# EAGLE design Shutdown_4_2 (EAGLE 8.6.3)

## Sheet 1 of 5: Power
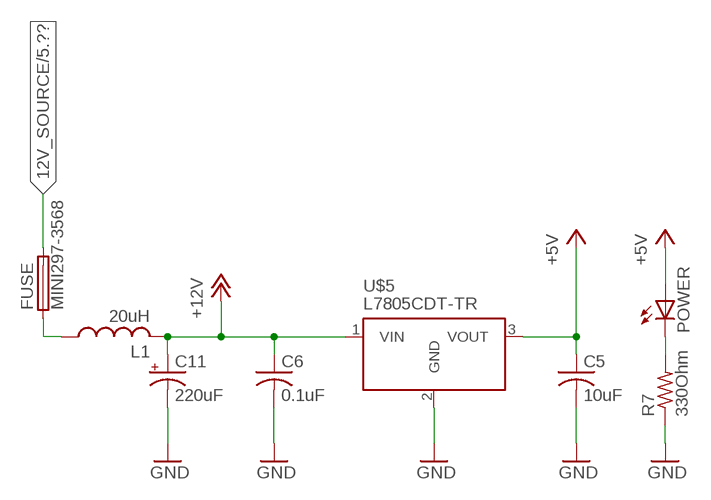
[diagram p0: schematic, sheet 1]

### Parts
C5  10uF  C0805  [C0805]
C6  0.1uF  C0805  [C0805]
C11  220uF  CPOL-USUD-6,3X7,7  [UD-6,3X7,7_NICHICON]
FUSE  MINI297-3568  [3568]
L1  20uH  MSS7348  [MSS7348]
POWER  LED0805  [LED0805]
R7  330Ohm  R0805  [R0805]
U$5  L7805CDT-TR  [DPACK]

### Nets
12V_SOURCE: FUSE.P$2 FUSE.P$3 ; also sheet 5
+5V: C5.1 POWER.1(A) U$5.3(VOUT) ; also sheet 2,3,5
+12V: C6.1 C11.+ L1.P$2 U$5.1(VIN) ; also sheet 3,4
GND: C5.2 C6.2 C11.- R7.1 U$5.2(GND) ; also sheet 2,3,4,5
N$2: FUSE.P$1 FUSE.P$4 L1.P$1
N$4: POWER.2(C) R7.2

## Sheet 2 of 5: Micro and CAN
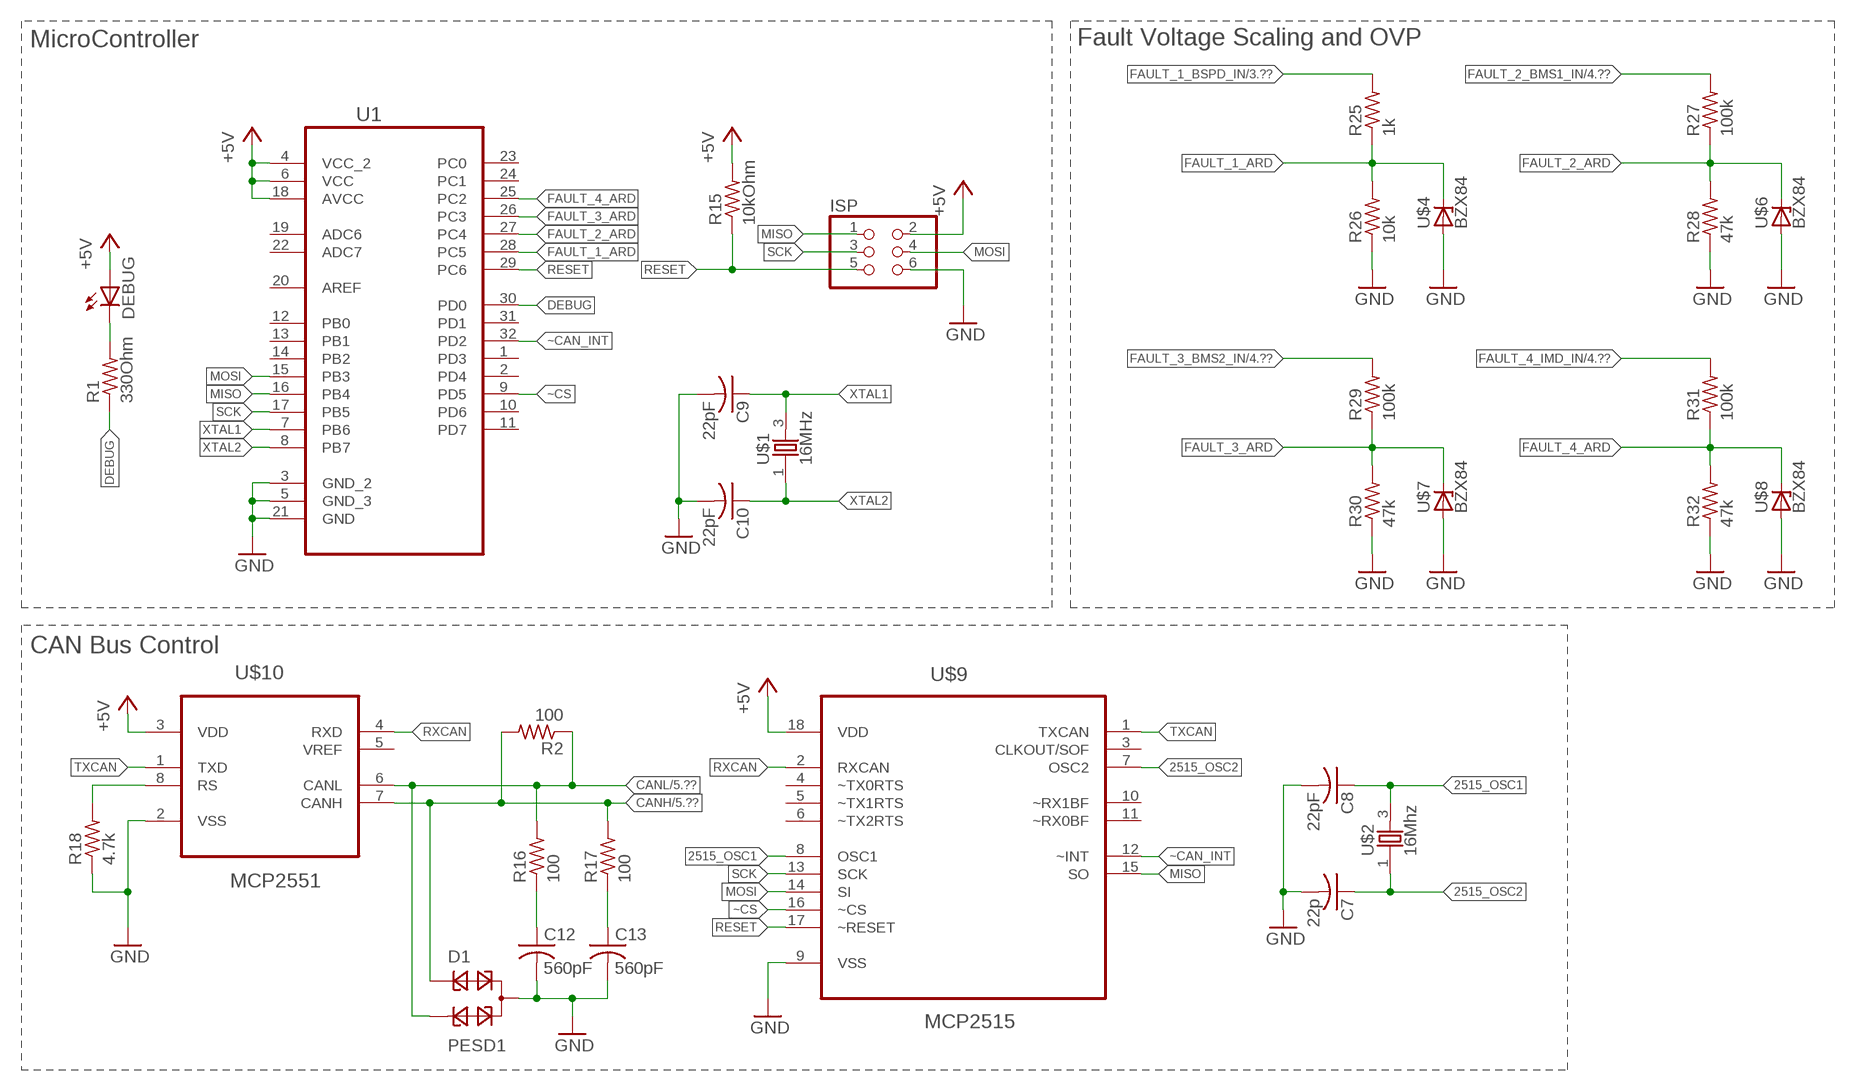
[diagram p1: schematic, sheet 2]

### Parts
C7  22p  C0805  [C0805]
C8  22pF  C0805  [C0805]
C9  22pF  C0805  [C0805]
C10  22pF  C0805  [C0805]
C12  560pF  C0805  [C0805]
C13  560pF  C0805  [C0805]
D1  PESD1  PESD1CAN  [SOT23]
DEBUG  LED0805  [LED0805]
ISP  PINHD-2X3  [2X03]
R1  330Ohm  R0805  [R0805]
R2  100  R0805  [R0805]
R15  10kOhm  R0805  [R0805]
R16  100  R0805  [R0805]
R17  100  R0805  [R0805]
R18  4.7k  R0805  [R0805]
R25  1k  R0805  [R0805]
R26  10k  R0805  [R0805]
R27  100k  R0805  [R0805]
R28  47k  R0805  [R0805]
R29  100k  R0805  [R0805]
R30  47k  R0805  [R0805]
R31  100k  R0805  [R0805]
R32  47k  R0805  [R0805]
U1  ATMEGA328P-AU  [QFP80P900X900X120-32N]
U$1  16MHz  406CYRYSTAL  [CTS406]
U$2  16Mhz  406CYRYSTAL  [CTS406]
U$4  BZX84  [SOT23]
U$6  BZX84  [SOT23]
U$7  BZX84  [SOT23]
U$8  BZX84  [SOT23]
U$9  MCP2515  MCP2515-I/SO  [SOIC127P1034X264-18N]
U$10  MCP2551  MCP2551-I/SN  [SOIC127P600X175-8N]

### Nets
2515_OSC1: C8.1 U$2.3 U$9.8(OSC1)
2515_OSC2: C7.1 U$2.1 U$9.7(OSC2)
+5V: DEBUG.1(A) ISP.2 R15.2 U1.4(VCC_2) U1.6(VCC) U1.18(AVCC) U$9.18(VDD) U$10.3(VDD) ; also sheet 1,3,5
CANH: D1.1 R2.2 R17.2 U$10.7(CANH) ; also sheet 5
CANL: D1.2 R2.1 R16.2 U$10.6(CANL) ; also sheet 5
DEBUG: R1.1 U1.30(PD0)
FAULT_1_ARD: R25.1 R26.2 U1.28(PC5) U$4.3(C)
FAULT_1_BSPD_IN: R25.2 ; also sheet 3,4
FAULT_2_ARD: R27.1 R28.2 U1.27(PC4) U$6.3(C)
FAULT_2_BMS1_IN: R27.2 ; also sheet 4,5
FAULT_3_ARD: R29.1 R30.2 U1.26(PC3) U$7.3(C)
FAULT_3_BMS2_IN: R29.2 ; also sheet 4,5
FAULT_4_ARD: R31.1 R32.2 U1.25(PC2) U$8.3(C)
FAULT_4_IMD_IN: R31.2 ; also sheet 4,5
GND: C7.2 C8.2 C9.2 C10.2 C12.2 C13.2 D1.3 ISP.6 R18.1 R26.1 R28.1 R30.1 R32.1 U1.3(GND_2) U1.5(GND_3) U1.21(GND) U$4.1(A) U$6.1(A) U$7.1(A) U$8.1(A) U$9.9(VSS) U$10.2(VSS) ; also sheet 1,3,4,5
MISO: ISP.1 U1.16(PB4) U$9.15(SO)
MOSI: ISP.4 U1.15(PB3) U$9.14(SI)
N$1: DEBUG.2(C) R1.2
N$12: C12.1 R16.1
N$13: C13.1 R17.1
N$14: R18.2 U$10.8(RS)
RESET: ISP.5 R15.1 U1.29(PC6) U$9.17(~RESET)
RXCAN: U$9.2(RXCAN) U$10.4(RXD)
SCK: ISP.3 U1.17(PB5) U$9.13(SCK)
TXCAN: U$9.1(TXCAN) U$10.1(TXD)
XTAL1: C9.1 U1.7(PB6) U$1.3
XTAL2: C10.1 U1.8(PB7) U$1.1
~CAN_INT: U1.32(PD2) U$9.12(~INT)
~CS: U1.9(PD5) U$9.16(~CS)
Unconnected: U1.1(PD3) U1.2(PD4) U1.10(PD6) U1.11(PD7) U1.12(PB0) U1.13(PB1) U1.14(PB2) U1.19(ADC6) U1.20(AREF) U1.22(ADC7) U1.23(PC0) U1.24(PC1) U1.31(PD1) U$9.3(CLKOUT/SOF) U$9.4(~TX0RTS) U$9.5(~TX1RTS) U$9.6(~TX2RTS) U$9.10(~RX1BF) U$9.11(~RX0BF) U$10.5(VREF)

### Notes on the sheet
- MicroController | Fault Voltage Scaling and OVP
- CAN Bus Control

## Sheet 3 of 5: BSPD Detection Circuit
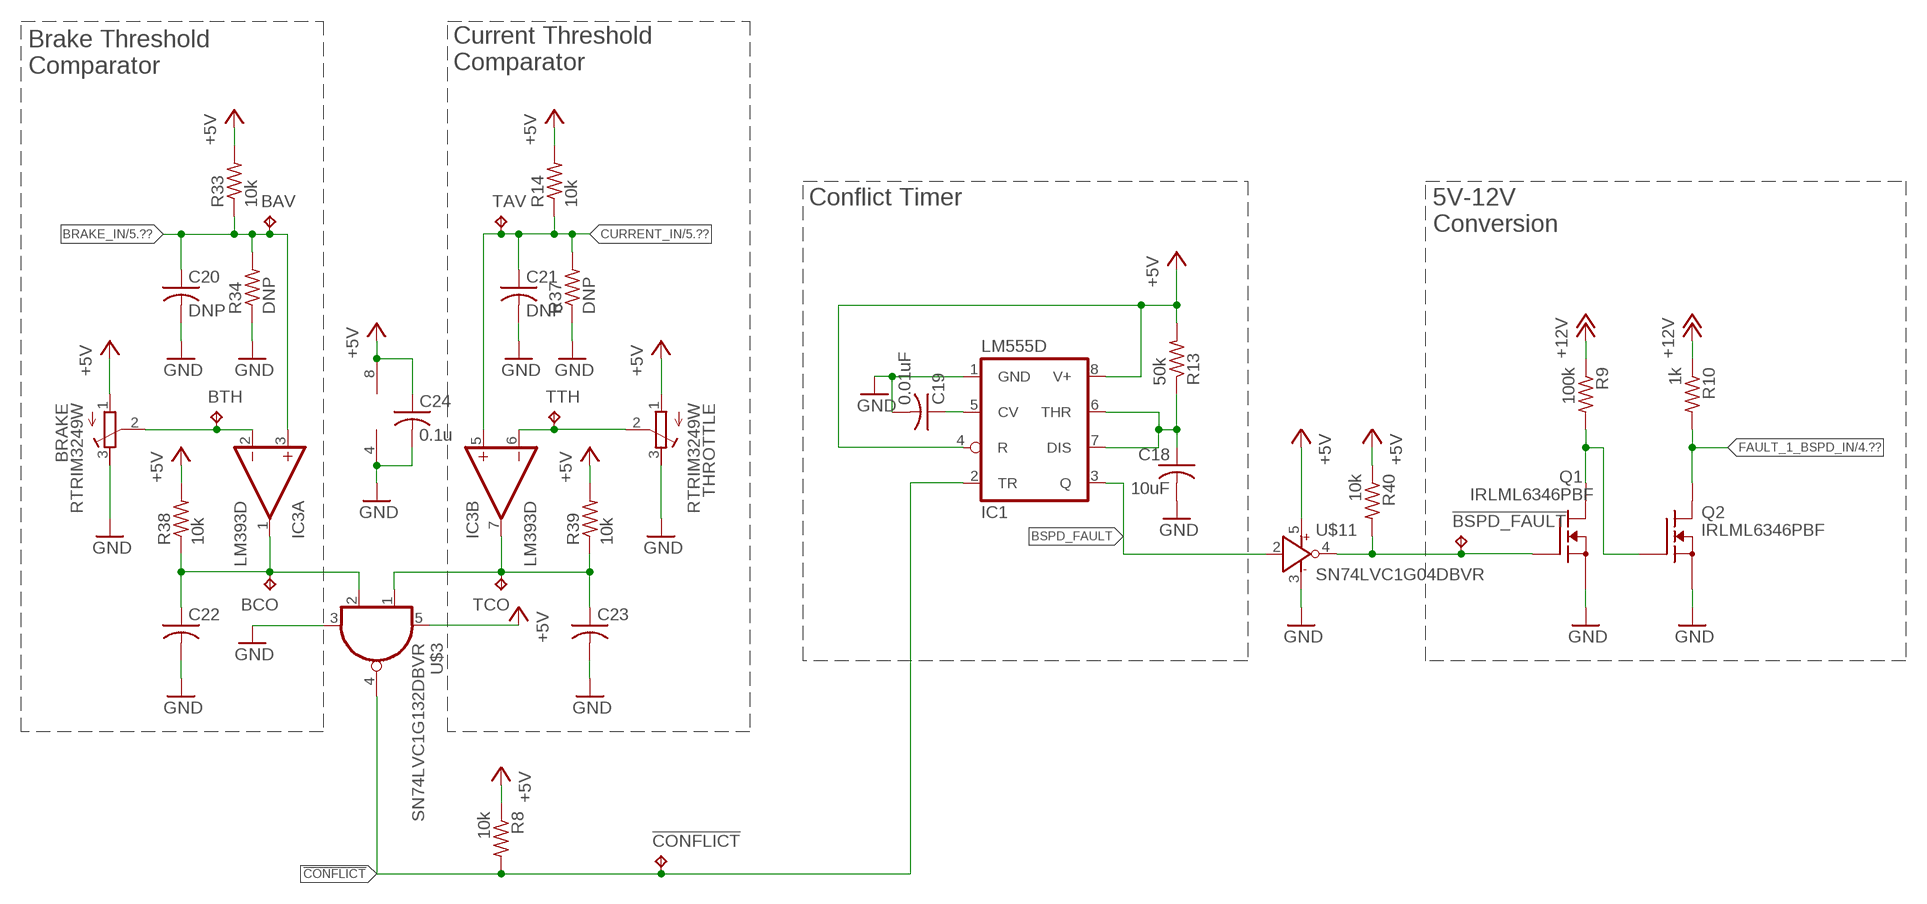
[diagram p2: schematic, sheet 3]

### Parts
!BSPD_FAULT  TPTP09R  [TP09R]
!CONFLICT  TPTP09R  [TP09R]
BAV  TPTP09R  [TP09R]
BCO  TPTP09R  [TP09R]
BRAKE  RTRIM3249W  [RTRIM3299W]
BTH  TPTP09R  [TP09R]
C18  10uF  C0805  [C0805]
C19  0.01uF  C0805  [C0805]
C20  DNP  C0805  [C0805]
C21  DNP  C0805  [C0805]
C22  C0805  [C0805]
C23  C0805  [C0805]
C24  0.1u  C0805  [C0805]
IC1  LM555D  [SO08]
IC3  LM393D  [SO08]
Q1  IRLML6346PBF  [SOT23]
Q2  IRLML6346PBF  [SOT23]
R8  10k  R0805  [R0805]
R9  100k  R0805  [R0805]
R10  1k  R0805  [R0805]
R13  50k  R0805  [R0805]
R14  10k  R0805  [R0805]
R33  10k  R0805  [R0805]
R34  DNP  R0805  [R0805]
R37  DNP  R0805  [R0805]
R38  10k  R0805  [R0805]
R39  10k  R0805  [R0805]
R40  10k  R0805  [R0805]
TAV  TPTP09R  [TP09R]
TCO  TPTP09R  [TP09R]
THROTTLE  RTRIM3249W  [RTRIM3299W]
TTH  TPTP09R  [TP09R]
U$3  SN74LVC1G132DBVR  [SOT23-5L]
U$11  SN74LVC1G04DBVR  [SOT23-5L]

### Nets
!CONFLICT: !CONFLICT.TP IC1.2(TR) R8.2 U$3.4(Y)
+5V: BRAKE.1(A) C24.1 IC1.4(R) IC1.8(V+) IC3.8(P:V+) R8.1 R13.2 R14.2 R33.2 R38.2 R39.2 R40.1 THROTTLE.1(A) U$3.5(V+) U$11.5(V+) ; also sheet 1,2,5
+12V: R9.1 R10.1 ; also sheet 1,4
BRAKE_IN: BAV.TP C20.1 IC3.3(A:+IN) R33.1 R34.2 ; also sheet 5
BSPD_FAULT: IC1.3(Q) U$11.2(A)
CURRENT_IN: C21.1 IC3.5(B:+IN) R14.1 R37.2 TAV.TP ; also sheet 5
FAULT_1_BSPD_IN: Q2.3(D) R10.2 ; also sheet 2,4
GND: BRAKE.3(E) C18.2 C19.2 C20.2 C21.2 C22.2 C23.2 C24.2 IC1.1(GND) IC3.4(P:V-) Q1.2(S) Q2.2(S) R34.1 R37.1 THROTTLE.3(E) U$3.3(GND) U$11.3(GND) ; also sheet 1,2,4,5
N$3: C23.1 IC3.7(B:OUT) R39.1 TCO.TP U$3.1(A)
N$5: BCO.TP C22.1 IC3.1(A:OUT) R38.1 U$3.2(B)
N$6: BRAKE.2(S) BTH.TP IC3.2(A:-IN)
N$7: !BSPD_FAULT.TP Q1.1(G) R40.2 U$11.4(Y)
N$10: C18.1 IC1.6(THR) IC1.7(DIS) R13.1
N$11: C19.1 IC1.5(CV)
N$15: Q1.3(D) Q2.1(G) R9.2
N$16: IC3.6(B:-IN) THROTTLE.2(S) TTH.TP

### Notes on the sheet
- Current Threshold
  Comparator
- Brake Threshold
  Comparator
- Conflict Timer
- 5V-12V
  Conversion

## Sheet 4 of 5: AIR Shutdown Relays + Fault Indication
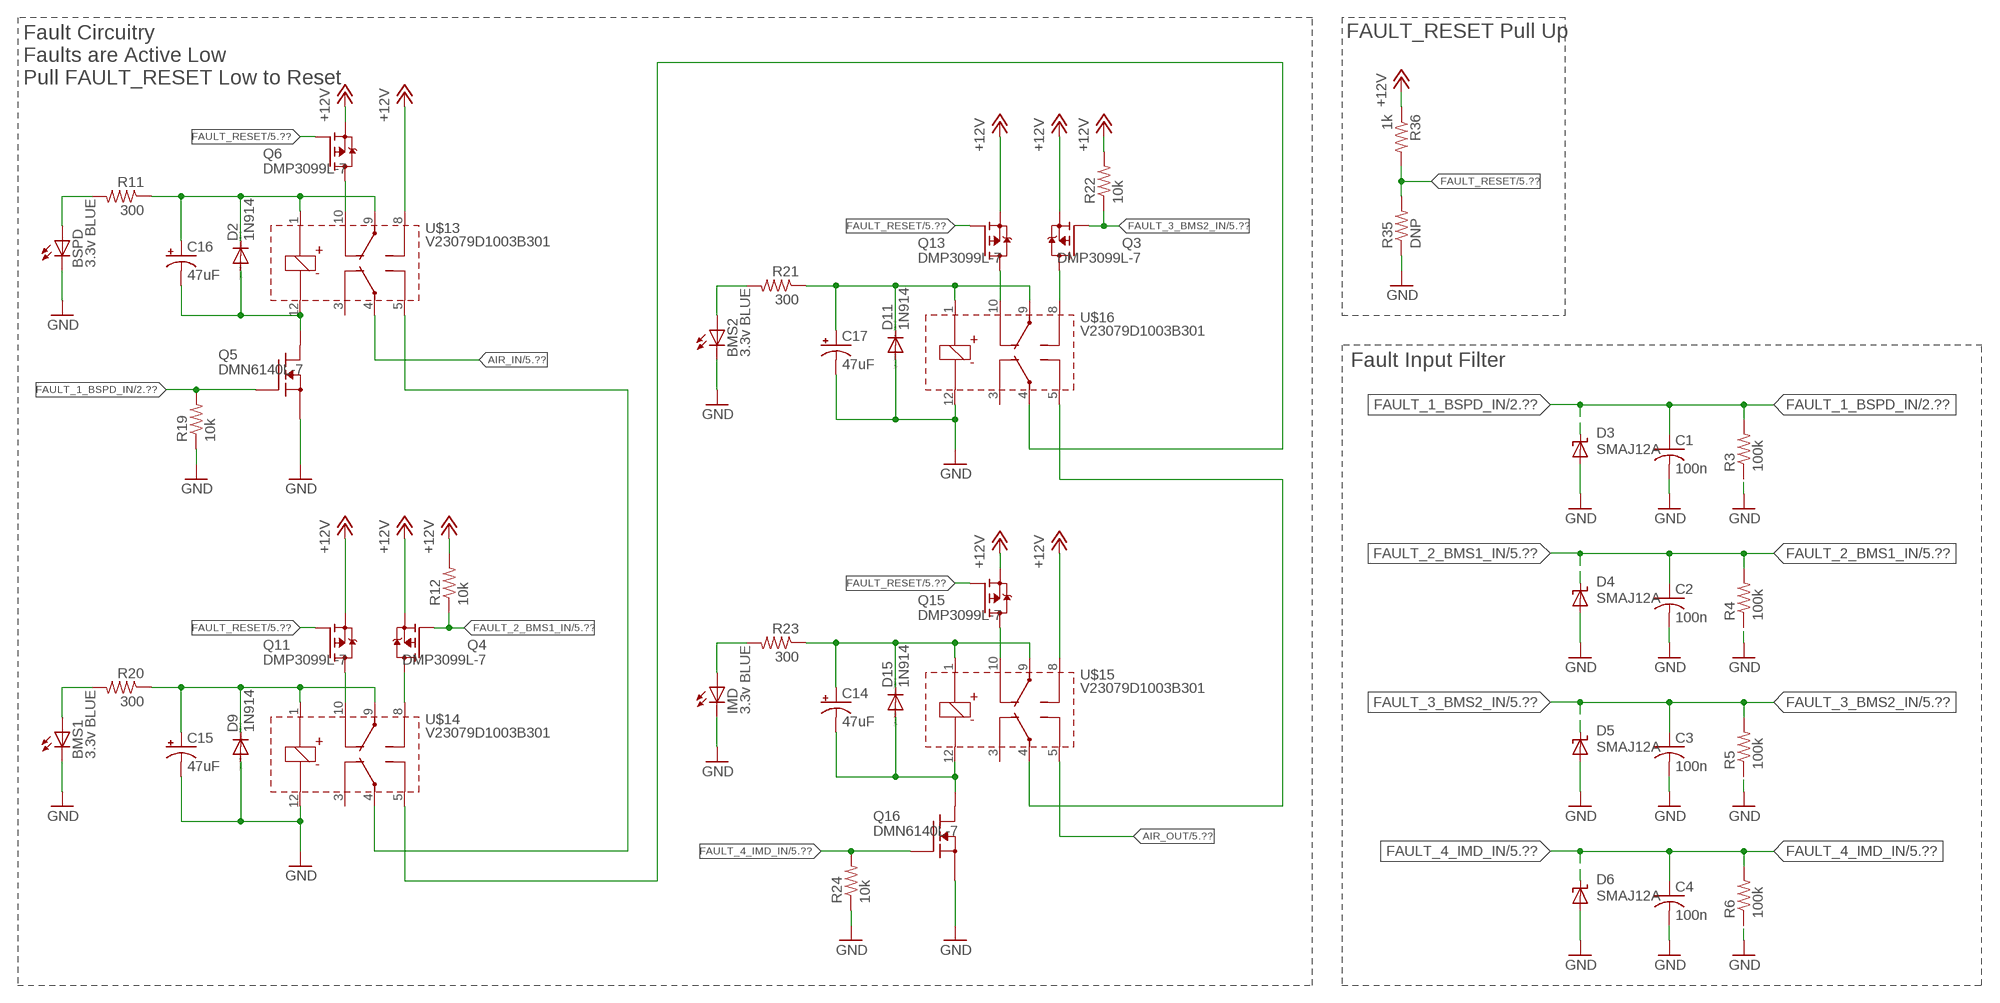
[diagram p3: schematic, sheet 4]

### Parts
BMS1  3.3v BLUE  LEDCHIPLED_0805  [CHIPLED_0805]
BMS2  3.3v BLUE  LEDCHIPLED_0805  [CHIPLED_0805]
BSPD  3.3v BLUE  LEDCHIPLED_0805  [CHIPLED_0805]
C1  100n  C0805  [C0805]
C2  100n  C0805  [C0805]
C3  100n  C0805  [C0805]
C4  100n  C0805  [C0805]
C14  47uF  CPOL-USUD-6,3X5,8  [UD-6,3X5,8_NICHICON]
C15  47uF  CPOL-USUD-6,3X5,8  [UD-6,3X5,8_NICHICON]
C16  47uF  CPOL-USUD-6,3X5,8  [UD-6,3X5,8_NICHICON]
C17  47uF  CPOL-USUD-6,3X5,8  [UD-6,3X5,8_NICHICON]
D2  1N914  [SOD323-F]
D3  SMAJ12A  [DO-214AC]
D4  SMAJ12A  [DO-214AC]
D5  SMAJ12A  [DO-214AC]
D6  SMAJ12A  [DO-214AC]
D9  1N914  [SOD323-F]
D11  1N914  [SOD323-F]
D15  1N914  [SOD323-F]
IMD  3.3v BLUE  LEDCHIPLED_0805  [CHIPLED_0805]
Q3  DMP3099L-7  [SOT23]
Q4  DMP3099L-7  [SOT23]
Q5  DMN6140L-7  [SOT23]
Q6  DMP3099L-7  [SOT23]
Q11  DMP3099L-7  [SOT23]
Q13  DMP3099L-7  [SOT23]
Q15  DMP3099L-7  [SOT23]
Q16  DMN6140L-7  [SOT23]
R3  100k  R0805  [R0805]
R4  100k  R0805  [R0805]
R5  100k  R0805  [R0805]
R6  100k  R0805  [R0805]
R11  300  R0805  [R0805]
R12  10k  R0805  [R0805]
R19  10k  R0805  [R0805]
R20  300  R0805  [R0805]
R21  300  R0805  [R0805]
R22  10k  R0805  [R0805]
R23  300  R0805  [R0805]
R24  10k  R0805  [R0805]
R35  DNP  R0805  [R0805]
R36  1k  R0805  [R0805]
U$13  V23079D1003B301  [DPDT_2C]
U$14  V23079D1003B301  [DPDT_2C]
U$15  V23079D1003B301  [DPDT_2C]
U$16  V23079D1003B301  [DPDT_2C]

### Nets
+12V: Q3.2(S) Q4.2(S) Q6.2(S) Q11.2(S) Q13.2(S) Q15.2(S) R12.2 R22.2 R36.1 U$13.8(2_ACTIVE) U$15.8(2_ACTIVE) ; also sheet 1,3
AIR_IN: U$13.4(1_CENTER) ; also sheet 5
AIR_OUT: U$15.5(1_ACTIVE) ; also sheet 5
BMS1_FAULT_INDICATOR: C15.+ D9.C R20.1 U$14.1(COIL+) U$14.9(2_CENTER)
BMS2_FAULT_INDICATOR: C17.+ D11.C R21.1 U$16.1(COIL+) U$16.9(2_CENTER)
BSPD_FAULT_INDICATOR: C16.+ D2.C R11.1 U$13.1(COIL+) U$13.9(2_CENTER)
FAULT_1_BSPD_IN: C1.1 D3.C Q5.1(G) R3.2 R19.2 ; also sheet 2,3
FAULT_2_BMS1_IN: C2.1 D4.C Q4.1(G) R4.2 R12.1 ; also sheet 2,5
FAULT_3_BMS2_IN: C3.1 D5.C Q3.1(G) R5.2 R22.1 ; also sheet 2,5
FAULT_4_IMD_IN: C4.1 D6.C Q16.1(G) R6.2 R24.2 ; also sheet 2,5
FAULT_RESET: Q6.1(G) Q11.1(G) Q13.1(G) Q15.1(G) R35.2 R36.2 ; also sheet 5
GND: BMS1.C BMS2.C BSPD.C C1.2 C2.2 C3.2 C4.2 C15.- C17.- D3.A D4.A D5.A D6.A D9.A D11.A IMD.C Q5.2(S) Q16.2(S) R3.1 R4.1 R5.1 R6.1 R19.1 R24.1 R35.1 U$14.12(COIL-) U$16.12(COIL-) ; also sheet 1,2,3,5
IMD_FAULT_INDICATOR: C14.+ D15.C R23.1 U$15.1(COIL+) U$15.9(2_CENTER)
N$8: BSPD.A R11.2
N$9: Q4.3(D) U$14.8(2_ACTIVE)
N$18: Q3.3(D) U$16.8(2_ACTIVE)
N$27: U$13.5(1_ACTIVE) U$14.4(1_CENTER)
N$28: Q6.3(D) U$13.10(2_REST)
N$31: U$14.5(1_ACTIVE) U$16.4(1_CENTER)
N$32: C16.- D2.A Q5.3(D) U$13.12(COIL-)
N$34: BMS1.A R20.2
N$35: Q11.3(D) U$14.10(2_REST)
N$36: U$15.4(1_CENTER) U$16.5(1_ACTIVE)
N$37: BMS2.A R21.2
N$38: Q13.3(D) U$16.10(2_REST)
N$42: IMD.A R23.2
N$43: Q15.3(D) U$15.10(2_REST)
N$44: C14.- D15.A Q16.3(D) U$15.12(COIL-)
Unconnected: U$13.3(1_REST) U$14.3(1_REST) U$15.3(1_REST) U$16.3(1_REST)

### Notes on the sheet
- FAULT_RESET Pull Up
- Fault Circuitry
  Faults are Active Low
  Pull FAULT_RESET Low to Reset
- Fault Input Filter

## Sheet 5 of 5: Connector
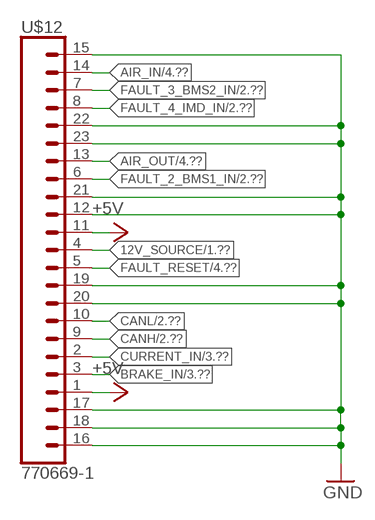
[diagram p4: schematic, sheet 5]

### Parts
U$12  770669-1  [770669-1]

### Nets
12V_SOURCE: U$12.4 ; also sheet 1
+5V: U$12.1 U$12.11 ; also sheet 1,2,3
AIR_IN: U$12.14 ; also sheet 4
AIR_OUT: U$12.13 ; also sheet 4
BRAKE_IN: U$12.3 ; also sheet 3
CANH: U$12.9 ; also sheet 2
CANL: U$12.10 ; also sheet 2
CURRENT_IN: U$12.2 ; also sheet 3
FAULT_2_BMS1_IN: U$12.6 ; also sheet 2,4
FAULT_3_BMS2_IN: U$12.7 ; also sheet 2,4
FAULT_4_IMD_IN: U$12.8 ; also sheet 2,4
FAULT_RESET: U$12.5 ; also sheet 4
GND: U$12.12 U$12.15 U$12.16 U$12.17 U$12.18 U$12.19 U$12.20 U$12.21 U$12.22 U$12.23 ; also sheet 1,2,3,4

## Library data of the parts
!BSPD_FAULT !CONFLICT BAV BCO BTH TAV TCO TTH = testpad:TP: Test pad
BMS1 BMS2 BSPD IMD = led:LED: LED
BRAKE THROTTLE = Resistors:RTRIM3249W
C1-C10 C12 C13 C18-C24 = Capacitors:C0805
C11 C14-C17 = rcl:CPOL-US: POLARIZED CAPACITOR, American symbol; SPICEPREFIX: C
D1 = diode:PESD1CAN: CAN bus ESD protection diode Source: http://www.nxp.com/documents/data_sheet/PESD1CAN.pdf
D2 D9 D11 D15 = Diodes:1N914
D3-D6 = Diodes:SMAJ12A
DEBUG POWER = LEDS:LED0805
FUSE = Fuse:MINI297-3568
IC1 = bspd2:*555: TIMER Changed DIP package to have round (not oval) pin pads http://www.ladyada.net/library/pcb/eaglelibrary.html
IC3 = IC's:LM393: COMPARATOR
ISP = pinhead:PINHD-2X3: PIN HEADER
L1 = Inductors:MSS7348
Q1 Q2 = TRANS:IRLML6346PBF: IRLML6346TRPBF Vgs(th) = 1.1V, Rds(on) = 63 mOhm, Vds(max) = 30V
Q3 Q4 Q6 Q11 Q13 Q15 = TRANS:DMP3099L-7: DMP3099L-7 P-Channel Vgs(th) = 2.1V, Rds(on) = 64 mohm, Vds(max) = 30V
Q5 Q16 = TRANS:DMN6140L-7: DMN6140L-7 Vgs(th) = 3V, Rds(on) = 140mOhm, Vds(max) = 60V
R1-R40 = Resistors:R0805
U1 = Atmel_By_element14_Batch_1-00:ATMEGA328P-AU: 8-bit Microcontroller with In-System Programmable Flash; MPN: ATMEGA328P-AU; OC_FARNELL: 1715486; OC_NEWARK: 14R4631; PACKAGE: TQFP-32; SUPPLIER: Atmel
U$1 U$2 = Display_Custom:406CYRYSTAL: Crystal Oscillator in 406 SMT Package
U$3 = Display_Custom:SN74LVC1G132DBVR: TI Single NAND SN74LVC1G132DBVR http://www.ti.com/lit/ds/symlink/sn74lvc1g132.pdf
U$4 U$6-U$8 = Diodes:BZX84: Zener Diode
U$5 = Display_Custom:L7805CDT-TR: ST - L78 L7805CDT-TR 5V 1.5A Linear Regulator
U$9 = Microchip_By_element14_Batch_1:MCP2515-I/SO: CAN Controller; MPN: MCP2515-I/SO; OC_FARNELL: 1292239; OC_NEWARK: 29H7136; PACKAGE: SOIC-18; SUPPLIER: Microchip
U$10 = Microchip_By_element14_Batch_1:MCP2551-I/SN: High-Speed CAN Transceiver; MPN: MCP2551-I/SN; OC_FARNELL: 9758569; OC_NEWARK: 69K7604; PACKAGE: SOIC-8; SUPPLIER: Microchip
U$11 = Display_Custom:SN74LVC1G04DBVR: TI Single Chip Inverter SN74LVC1G04DBVR http://www.ti.com/lit/ds/symlink/sn74lvc1g04.pdf
U$12 = IFE_AMPSEAL_Conn:770669-1: AMPSEAL 23pin Connector Ampseal 23-pin connector Model: 770669-1
U$13-U$16 = Display_Custom:V23079D1003B301: TE Connectivity Potter & Brumfield Relays V23079D1003B301 http://www.te.com/commerce/DocumentDelivery/DDEController?Action=srchrtrv&DocNm=108-98002&DocType=SS&DocLang=EN

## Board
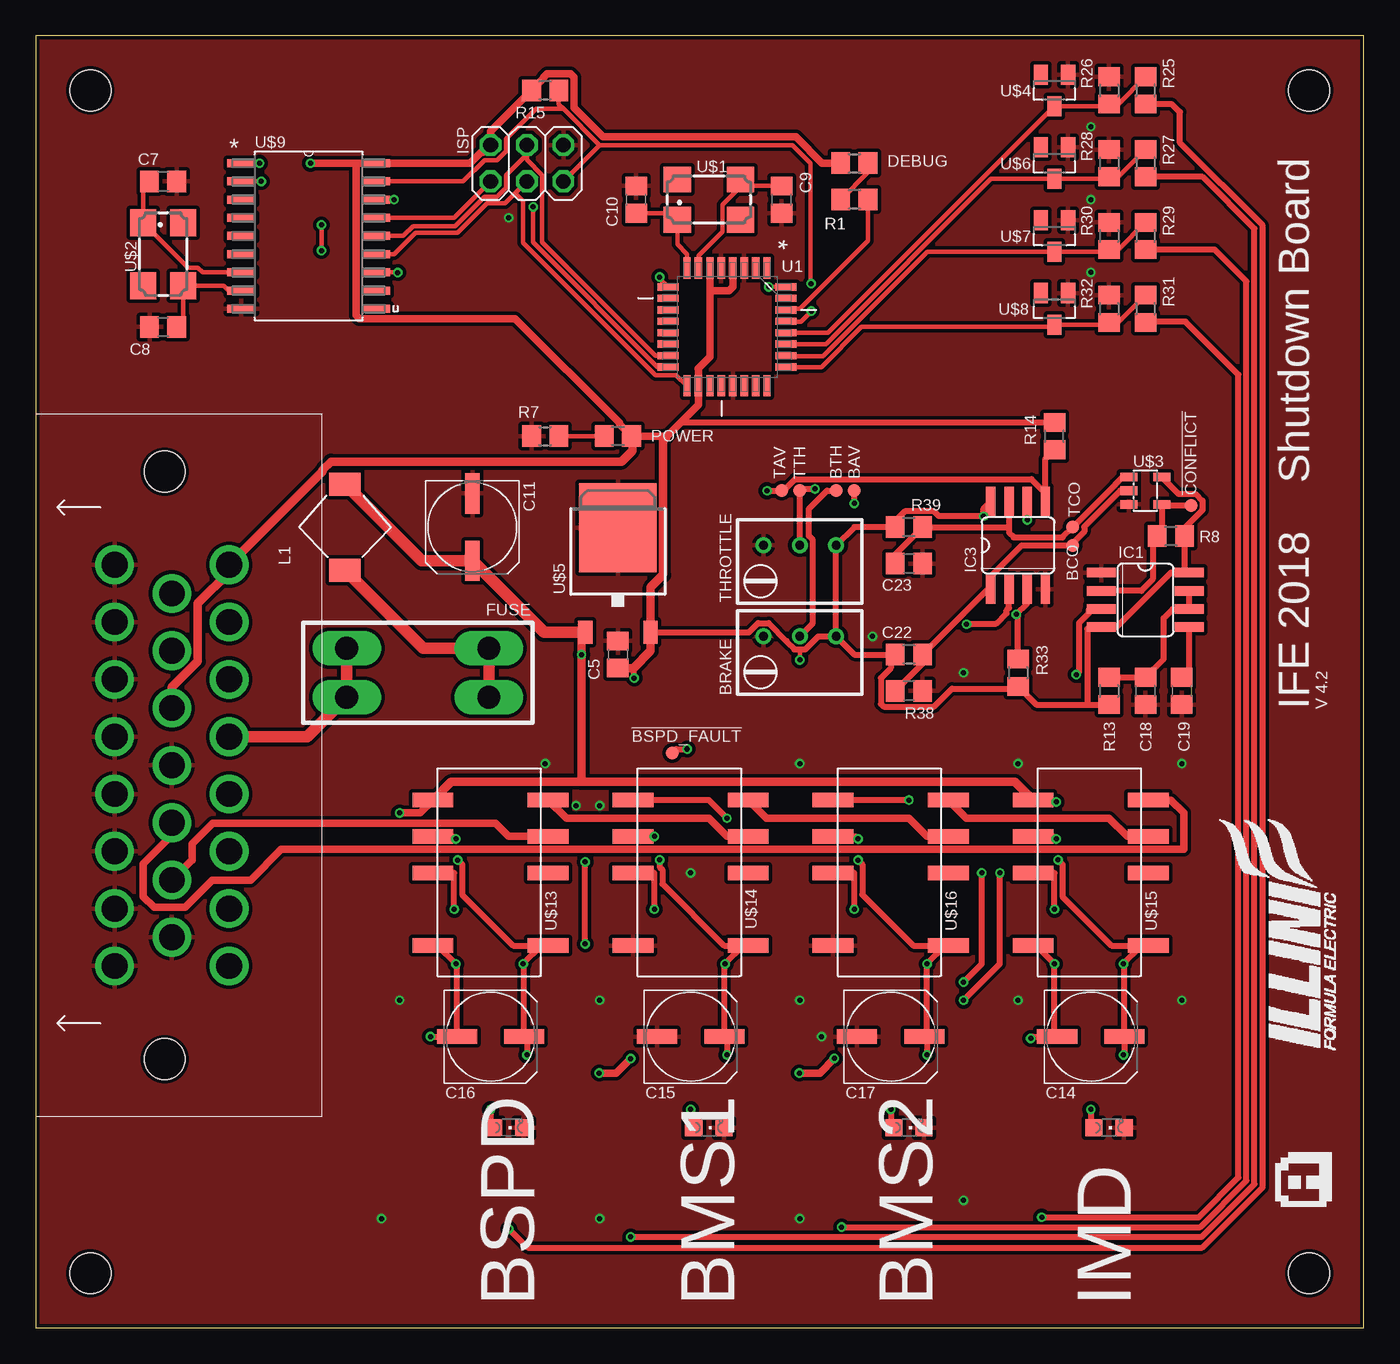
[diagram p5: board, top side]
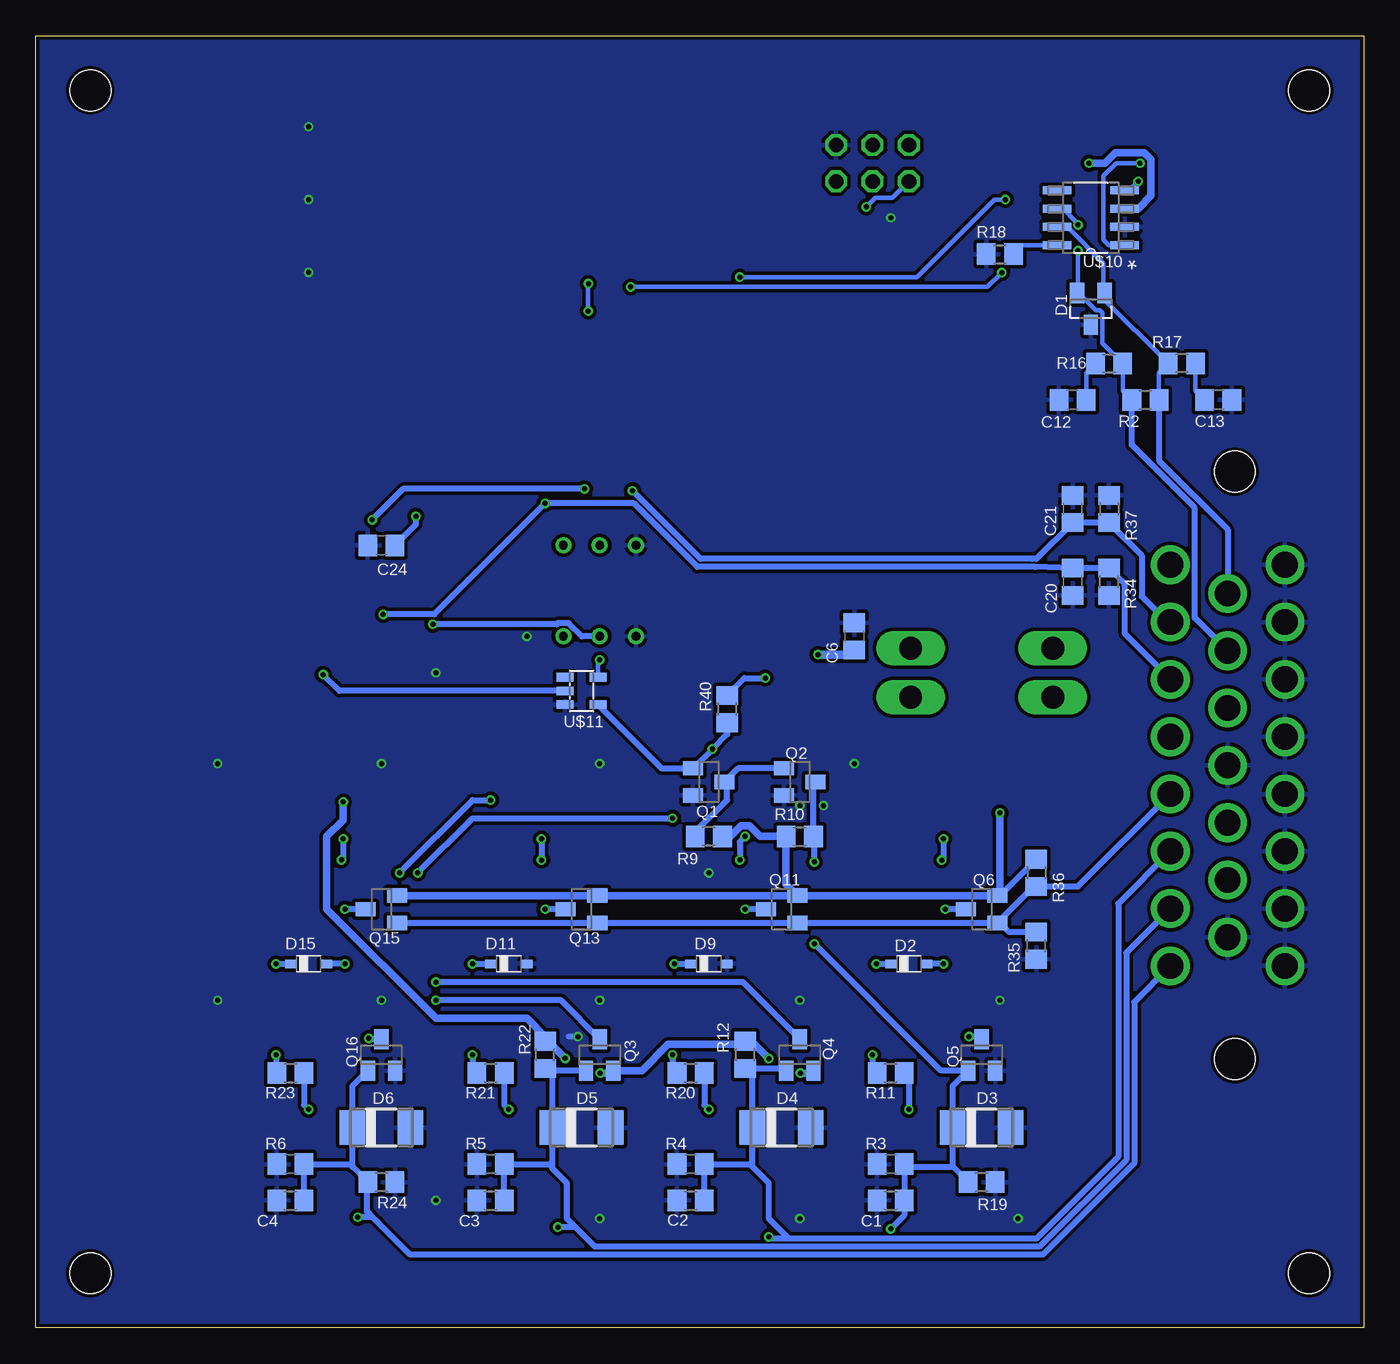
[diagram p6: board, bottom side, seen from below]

Size 92.71 x 90.17 mm. Coordinates in mm from the lower left corner, seen from the top.
Outline: 0,0 92.71,0 92.71,90.17 0,90.17 0,0
Copper layers (1*16): Top 0.035mm / dielectric 1.5mm / Bottom 0.035mm
Design rules "SeeedStudio_2layer_DRU_no_angle_20140221": minimum track width 6mil, minimum drill 12mil, track to track 6mil, track to pad 6mil, pad to pad 6mil, via to via 6mil, smd to smd 0mil, copper to edge 10mil, drill to drill 10mil, minimum pad ring 10mil, minimum via ring 6mil, stop-mask expansion 2mil, vias tented up to drill 100mil, thermal gap 10mil
Holes 2.84 mm at 3.81,3.81 3.81,86.36 88.9,86.36 88.9,3.81

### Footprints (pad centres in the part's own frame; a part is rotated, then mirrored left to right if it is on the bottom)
TP09R = smd 0.9 x 0.9: TP 0,0
CHIPLED_0805 = smd 1.2 x 1.2: A 0,-1.05; C 0,1.05
RTRIM3299W = drill 0.61: 1 1.27,-2.54; 2 1.27,0; 3 1.27,2.54
C0805 = smd 1.3 x 1.5: 1 -0.95,0; 2 0.95,0
UD-6,3X7,7_NICHICON = smd 2.8 x 1: + 2.35,0; - -2.35,0
UD-6,3X5,8_NICHICON = smd 2.8 x 1: + 2.35,0; - -2.35,0
SOT23 = smd 1 x 1.4: 1 -0.95,-1.1; 2 0.95,-1.1; 3 0,1.1
SOD323-F = smd 0.8 x 0.6: A 1.25,0; C -1.25,0
DO-214AC = smd 1.8 x 2.4: A 2.025,0; C -2.025,0
LED0805 = smd 1.3 x 1.5: 1 -0.95,0; 2 0.95,0
3568 = drill 1.6 long: P$1 -4.96,1.7; P$2 4.96,1.7; P$3 4.96,-1.7; P$4 -4.96,-1.7
SO08 = smd 0.66 x 2.032: 1 -1.905,-3.073; 2 -0.635,-3.073; 3 0.635,-3.073; 4 1.905,-3.073; 5 1.905,3.073; 6 0.635,3.073; 7 -0.635,3.073; 8 -1.905,3.073
2X03 = drill 1.016 octagon: 1 -2.54,-1.27; 2 -2.54,1.27; 3 0,-1.27; 4 0,1.27; 5 2.54,-1.27; 6 2.54,1.27
MSS7348 = smd 1.6 x 2.2: P$1 -3,0; P$2 3,0
R0805 = smd 1.3 x 1.5: 1 -0.95,0; 2 0.95,0
QFP80P900X900X120-32N = smd 1.473 x 0.508: 1 -4.115,2.794; 2 -4.115,2.007; 3 -4.115,1.194; 4 -4.115,0.406; 5 -4.115,-0.406; 6 -4.115,-1.194; 7 -4.115,-2.007; 8 -4.115,-2.794; 17 4.115,-2.794; 18 4.115,-2.007; 19 4.115,-1.194; 20 4.115,-0.406; 21 4.115,0.406; 22 4.115,1.194; 23 4.115,2.007; 24 4.115,2.794 | smd 0.508 x 1.473: 9 -2.794,-4.115; 10 -2.007,-4.115; 11 -1.194,-4.115; 12 -0.406,-4.115; 13 0.406,-4.115; 14 1.194,-4.115; 15 2.007,-4.115; 16 2.794,-4.115; 25 2.794,4.115; 26 2.007,4.115; 27 1.194,4.115; 28 0.406,4.115; 29 -0.406,4.115; 30 -1.194,4.115; 31 -2.007,4.115; 32 -2.794,4.115
CTS406 = smd 1.9 x 1.8: 1 -2.2,-1.4; 2 2.2,-1.4; 3 2.2,1.4; 4 -2.2,1.4
SOT23-5L = smd 0.6 x 1.2: 1 -0.95,-1.15; 2 0,-1.15; 3 0.95,-1.15; 4 0.95,1.15; 5 -0.95,1.15
DPACK = smd 1 x 1.6: 1 -2.28,-4.8; 3 2.28,-4.8 | smd 5.4 x 6.2: 2 0,2.5
SOIC127P1034X264-18N = smd 1.981 x 0.559: 1 -4.699,5.08; 2 -4.699,3.81; 3 -4.699,2.54; 4 -4.699,1.27; 5 -4.699,0; 6 -4.699,-1.27; 7 -4.699,-2.54; 8 -4.699,-3.81; 9 -4.699,-5.08; 10 4.699,-5.08; 11 4.699,-3.81; 12 4.699,-2.54; 13 4.699,-1.27; 14 4.699,0; 15 4.699,1.27; 16 4.699,2.54; 17 4.699,3.81; 18 4.699,5.08
SOIC127P600X175-8N = smd 1.981 x 0.559: 1 -2.362,1.905; 2 -2.362,0.635; 3 -2.362,-0.635; 4 -2.362,-1.905; 5 2.362,-1.905; 6 2.362,-0.635; 7 2.362,0.635; 8 2.362,1.905
770669-1 = drill 1.8: 1 10.5,13.5; 2 14.5,13.5; 3 18.5,13.5; 4 22.5,13.5; 5 26.5,13.5; 6 30.5,13.5; 7 34.5,13.5; 8 38.5,13.5; 9 12.5,9.5; 10 16.5,9.5; 11 20.5,9.5; 12 24.5,9.5; 13 28.5,9.5; 14 32.5,9.5; 15 36.5,9.5; 16 10.5,5.5; 17 14.5,5.5; 18 18.5,5.5; 19 22.5,5.5; 20 26.5,5.5; 21 30.5,5.5; 22 34.5,5.5; 23 38.5,5.5 | hole 2.85: 4,9; 45,9
DPDT_2C = smd 1 x 2.85: 1 -5.08,-4.025; 3 0,-4.025; 4 2.54,-4.025; 5 5.08,-4.025; 8 5.08,4.025; 9 2.54,4.025; 10 0,4.025; 12 -5.08,4.025

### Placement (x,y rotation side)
!BSPD_FAULT  44.45,40.13 0 top
!CONFLICT  80.64,57.4 0 top
BAV  57.15,58.42 0 top
BCO  72.39,54.61 0 top
BMS1  46.99,13.97 270 top
BMS2  60.96,13.97 270 top
BRAKE  53.34,46.99 90 top
BSPD  33.02,13.97 270 top
BTH  55.88,58.42 0 top
C1  33.02,11.43 180 bottom
C2  46.99,11.43 180 bottom
C3  60.96,11.43 180 bottom
C4  74.93,11.43 180 bottom
C5  40.64,46.99 90 top
C6  35.56,48.26 90 bottom
C7  8.89,80.01 0 top
C8  8.89,69.85 180 top
C9  52.07,78.74 270 top
C10  41.91,78.74 90 top
C11  30.48,55.88 270 top
C12  20.32,64.77 180 bottom
C13  10.16,64.77 0 bottom
C14  73.66,20.32 0 top
C15  45.72,20.32 0 top
C16  31.75,20.32 0 top
C17  59.69,20.32 0 top
C18  77.47,44.45 270 top
C19  80.01,44.45 270 top
C20  20.32,52.07 270 bottom
C21  20.32,57.15 90 bottom
C22  60.96,44.45 0 top
C23  60.96,53.34 0 top
C24  68.58,54.61 180 bottom
D1  19.05,71.12 180 bottom
D2  31.75,25.4 0 bottom
D3  26.67,13.97 0 bottom
D4  40.64,13.97 0 bottom
D5  54.61,13.97 0 bottom
D6  68.58,13.97 0 bottom
D9  45.72,25.4 0 bottom
D11  59.69,25.4 0 bottom
D15  73.66,25.4 0 bottom
DEBUG  57.15,81.28 0 top
FUSE  26.67,45.72 180 top
IC1  77.47,50.8 270 top
IC3  68.58,54.61 0 top
IMD  74.93,13.97 270 top
ISP  34.29,81.28 0 top
L1  21.59,55.88 90 top
POWER  40.64,62.23 180 top
Q1  45.72,38.1 270 bottom
Q2  39.37,38.1 270 bottom
Q3  53.34,19.05 0 bottom
Q4  39.37,19.05 0 bottom
Q5  26.67,19.05 0 bottom
Q6  26.67,29.21 90 bottom
Q11  40.64,29.21 90 bottom
Q13  54.61,29.21 90 bottom
Q15  68.58,29.21 90 bottom
Q16  68.58,19.05 0 bottom
R1  57.15,78.74 180 top
R2  15.24,64.77 0 bottom
R3  33.02,8.89 0 bottom
R4  46.99,8.89 0 bottom
R5  60.96,8.89 0 bottom
R6  74.93,8.89 0 bottom
R7  35.56,62.23 0 top
R8  79.25,55.24 180 top
R9  45.72,34.29 180 bottom
R10  39.37,34.29 0 bottom
R11  33.02,17.78 0 bottom
R12  43.18,19.05 90 bottom
R13  74.93,44.45 270 top
R14  71.12,62.23 90 top
R15  35.56,86.36 180 top
R16  17.78,67.31 0 bottom
R17  12.7,67.31 180 bottom
R18  25.4,74.93 0 bottom
R19  26.67,10.16 180 bottom
R20  46.99,17.78 0 bottom
R21  60.96,17.78 0 bottom
R22  57.15,19.05 90 bottom
R23  74.93,17.78 0 bottom
R24  68.58,10.16 180 bottom
R25  77.47,86.36 270 top
R26  74.93,86.36 270 top
R27  77.47,81.28 270 top
R28  74.93,81.28 270 top
R29  77.47,76.2 270 top
R30  74.93,76.2 270 top
R31  77.47,71.12 270 top
R32  74.93,71.12 270 top
R33  68.58,45.72 270 top
R34  17.78,52.07 90 bottom
R35  22.86,26.67 90 bottom
R36  22.86,31.75 270 bottom
R37  17.78,57.15 270 bottom
R38  60.96,46.99 180 top
R39  60.96,55.88 180 top
R40  44.45,43.18 270 bottom
TAV  52.07,58.42 0 top
TCO  72.39,55.88 0 top
THROTTLE  53.34,53.34 90 top
TTH  53.34,58.42 0 top
U1  48.26,69.85 270 top
U$1  46.99,78.74 0 top
U$2  8.89,74.93 270 top
U$3  77.47,58.42 270 top
U$4  71.12,86.36 180 top
U$5  40.64,53.34 0 top
U$6  71.12,81.28 180 top
U$7  71.12,76.2 180 top
U$8  71.12,71.12 180 top
U$9  19.05,76.2 0 top
U$10  19.05,77.47 180 bottom
U$11  54.61,44.45 270 bottom
U$12  0,63.75 270 top
U$13  31.75,31.75 90 top
U$14  45.72,31.75 90 top
U$15  73.66,31.75 90 top
U$16  59.69,31.75 90 top

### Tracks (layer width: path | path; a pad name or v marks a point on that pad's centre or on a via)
12V_SOURCE
  Top 0.813: FUSE.P$3 FUSE.P$2 18.94,41.25 U$12.4
2515_OSC1
  Top 0.305: U$9.8 13.46,72.39 13.12,72.73 U$2.3 10.29,70.3 C8.1
2515_OSC2
  Top 0.305: C7.1 7.49,79.56 U$2.1 10.63,73.98 11.32,73.98 11.64,73.66 U$9.7
!CONFLICT
  Top 0.406: !CONFLICT.TP 78.69,57.4 U$3.4 78.62,55.57 R8.2 77.98,54.92 77.98,52.23 77.19,51.44 IC1.2
+5V  (via drill 0.35)
  Top 0.305: v53.34,46.61 53.34,47.35
  Top 0.406: BRAKE.1 54.63,48.26 53.72,47.35 53.34,47.35 52.96,47.35 52.43,47.88 52.43,47.93 51.18,49.17 50.42,49.17 49.79,48.54 U$5.3 | BRAKE.1 THROTTLE.1 57.15,55.88 59.56,55.88 | BRAKE.1 57.15,46.99 59.69,46.99 | 59.69,46.99 R38.2 | R33.2 68.74,44.61 | 68.74,44.61 69.85,43.5 73.41,43.5 | 73.41,43.5 R13.2 | 73.41,43.5 73.41,48.77 73.53,48.9 IC1.4 75.44,48.9 79.25,52.7 80.14,52.7 | 45.92,64.06 45.91,64.07 | R14.2 45.02,63.18 44.9,63.06 | R39.2 59.56,55.88 | 80.14,52.7 IC1.8 | 80.14,52.7 80.2,52.77 R8.1 80.14,55.31 80.14,55.75 81.41,57.02 81.41,57.03 81.45,57.07 81.45,57.74 80.98,58.21 79.78,58.21 U$3.5 | v41.78,45.34 41.78,45.98 41.72,46.04 | IC3.8 66.17,57.17 v66.17,56.64 63.05,56.64 62.71,56.99 60.67,56.99 59.56,55.88 | 68.74,44.61 63.97,44.61 62.71,43.34 59.21,43.34 59,43.55 59,45.35 59.69,46.03 59.69,46.99
  Top 0.508: U1.6 47.07,72.39 | 47.07,72.39 47.07,67.77 46.23,66.93 46.25,66.9 U1.18 46.25,64.41 45.91,64.07 44.9,63.06 44.07,62.23 41.66,62.23 POWER.1 40.75,63.07 40.75,63.15 33.46,70.43 22.59,70.43 22.35,70.67 22.35,81.28 | 47.07,72.39 48.39,72.39 48.67,72.67 U1.4 | DEBUG.1 54.89,81.28 53.06,83.11 39.6,83.11 37.57,85.14 37.57,87.28 37.33,87.52 35.69,87.52 35.45,87.28 35.45,87.2 R15.2 31.75,83.5 ISP.2 31.24,82.04 31.09,82.04 30.32,81.28 U$9.18 22.35,81.28 | v19.18,81.28 22.35,81.28
  Top 0.61: 44.07,62.23 43.8,61.96 43.8,52.55 42.92,51.67 U$5.3 42.92,47.25 42.93,47.24 41.72,46.04 C5.1 | U$12.11 9.5,44.7 11.31,46.51 11.31,50.55 13.5,52.74 U$12.1 20.03,59.79 20.03,59.87 20.61,60.45 40.89,60.45 41.66,61.21 41.66,62.23
  Bottom 0.305: U$11.5 53.46,46.49 v53.34,46.61
  Bottom 0.406: R40.1 43.24,45.34 v41.78,45.34 | C24.1 66.17,56.07 v66.17,56.64
  Bottom 0.508: U$10.3 15.75,78.11 14.86,78.99 14.86,81.56 15.32,82.01 17.33,82.01 18.06,81.28 v19.18,81.28
+12V  (via drill 0.35)
  Top 0.508: U$13.8 26.82,35.93 v25.4,35.93 | v55.75,18.8 54.74,17.78 v53.31,17.78 | v41.53,18.78 40.53,17.78 v39.34,17.78 | U$15.8 69.76,36.7 v71.25,36.7
  Top 0.61: U$5.1 38.1,48.28 v38.1,46.99 38.1,38.1 | U$15.8 68.36,38.1 38.1,38.1 | U$13.8 29,38.1 38.1,38.1
  Top 0.813: L1.P$2 26.94,53.53 C11.+ 35.47,48.54 U$5.1
  Bottom 0.406: R36.1 23.75,31.81 23.76,31.81 25.4,30.16 Q6.2
  Bottom 0.508: Q6.2 Q11.2 | Q11.2 Q13.2 Q15.2 | R9.1 44.22,34.29 43.48,35.02 42.88,35.02 42.14,34.29 R10.1 40.32,30.94 Q11.2 | v25.4,35.93 25.4,30.16 | v55.75,18.8 56.96,20 R22.2 57.15,20.32 58.42,21.59 64.77,21.59 72.39,29.21 72.39,34.29 71.25,35.43 v71.25,36.7 | v53.31,17.78 52.56,17.78 Q3.2 50.4,17.95 48.56,19.78 43.4,19.78 R12.2 42.75,20 v41.53,18.78 | v39.34,17.78 38.59,17.78 Q4.2
  Bottom 0.61: v38.1,46.99 35.88,46.99 C6.1
AIR_IN
  Top 0.508: U$12.14 10.88,32.64 10.92,32.64 10.92,33.78 12.34,35.2 29.21,35.2 29.32,35.2 32.11,35.2 33.02,34.29 U$13.4
AIR_OUT
  Top 0.508: U$15.5 79.25,36.83 80.14,35.94 80.14,33.4 79.3,33.4 79.28,33.38 17.13,33.38 14.99,31.24 12.32,31.24 10.41,29.34 8.26,29.34 7.49,30.1 7.49,32.38 9.5,34.39 U$12.13
BMS1_FAULT_INDICATOR  (via drill 0.35)
  Top 0.406: v48.26,19.05 48.26,20.13 C15.+ 48.07,25.34 v48.13,25.4 49.4,26.67 | 49.4,26.67 U$14.1 | U$14.9 v43.18,34.29 | v43.56,32.65 43.56,32.16 43.74,31.98 43.74,30.99 48.06,26.67 49.4,26.67
  Bottom 0.406: v48.26,19.05 48.26,18.1 R20.1 | v48.13,25.4 D9.C | v43.18,34.29 43.56,33.91 v43.56,32.65
BMS2_FAULT_INDICATOR  (via drill 0.35)
  Top 0.406: 63.5,26.67 v62.23,25.4 62.23,20.51 C17.+ 62.23,20.13 v62.23,19.05 | 63.5,26.67 U$16.1 | U$16.9 57.23,34.29 v57.4,34.12 | v57.4,32.64 57.71,32.33 57.71,30.23 61.27,26.67 63.5,26.67
  Bottom 0.406: v62.23,25.4 D11.C | v62.23,19.05 62.23,18.1 R21.1 | v57.4,34.12 v57.4,32.64
BRAKE_IN  (via drill 0.35)
  Top 0.406: v57.15,57.53 BAV.TP | IC3.3 69.22,50.55 v68.45,49.78 68.58,49.66 R33.1
  Bottom 0.406: v68.45,49.78 64.9,49.78 v57.15,57.53 50.95,57.53 46.52,53.1 22.94,53.1 C20.1 R34.2 16.89,52.13 16.88,52.13 16.67,51.92 16.67,48.43 U$12.3
BSPD_FAULT  (via drill 0.35)
  Top 0.406: v72.64,45.59 72.85,45.8 72.85,49.2 73.53,49.88 73.53,50.16 IC1.3
  Bottom 0.406: U$11.2 71.5,44.45 v72.64,45.59
BSPD_FAULT_INDICATOR  (via drill 0.35)
  Top 0.406: v34.29,19.05 34.29,20.13 C16.+ 34.1,25.34 v34.04,25.4 35.31,26.67 | 35.31,26.67 U$13.1 | U$13.9 29.16,34.29 v29.34,34.12 | v29.46,32.64 29.77,32.33 29.77,30.23 33.33,26.67 35.31,26.67
  Bottom 0.406: v34.29,19.05 34.29,18.1 R11.1 | v34.04,25.4 D2.C | v29.34,34.12 29.34,32.77 v29.46,32.64
CANH
  Bottom 0.305: U$10.7 20.7,76.83 18.16,74.3 18.16,72.28 | 18.16,72.28 D1.1 | R2.2 14.29,66.67 R17.2 18.16,71.82 18.16,72.28
  Bottom 0.406: R2.2 14.29,60.52 9.5,55.73 U$12.9
CANL  (via drill 0.35)
  Top 0.305: v19.94,75.18 v19.94,76.97
  Bottom 0.305: v19.94,75.18 19.94,72.28 D1.2 19.9,72.22 18.7,71.03 18.42,71.03 18.25,70.85 18.25,68.72 R16.2 16.83,65.41 R2.1 | v19.94,76.97 20.12,77.14 20.12,77.24 20.98,78.11 U$10.6
  Bottom 0.406: U$12.10 11.79,49.55 11.79,57.23 16.19,61.63 R2.1
CURRENT_IN  (via drill 0.35)
  Top 0.406: v51.05,58.42 TAV.TP 52.2,58.42 53.01,59.23 69.52,59.23 70.33,58.42 70.48,58.42 | IC3.5 70.48,58.42 | 70.48,58.42 70.48,60.65 R14.1
  Bottom 0.406: v51.05,58.42 46.29,53.66 23.16,53.66 23.16,53.67 22.85,53.67 C21.1 R37.2 15.49,53.91 15.49,51.05 13.69,49.25 U$12.2
DEBUG
  Top 0.305: U1.30 52.45,71.12 53.34,71.12 58.1,75.88 R1.1
FAULT_1_ARD
  Top 0.305: R25.1 75.57,85.41 R26.2 74.78,85.26 U$4.3 55.3,69.44 U1.28
FAULT_1_BSPD_IN  (via drill 0.35)
  Top 0.406: v33.02,6.91 34.34,5.59 81.44,5.59 85.65,9.8 85.65,76.94 79.88,82.7 79.88,84.84 79.31,85.41 R25.2 | v38.35,26.8 v38.35,32.51
  Bottom 0.406: R19.2 28.7,11.23 | 28.7,11.23 D3.C 28.7,16.88 Q5.1 29.51,17.95 v38.35,26.8 | 28.7,11.23 31.88,11.23 C1.1 R3.2 32.07,7.86 v33.02,6.91 | 38.27,34.44 R10.2 | v38.35,32.51 38.35,34.22 R10.2 | 38.1,38.1 Q2.3 38.42,37.95 R10.2
FAULT_2_ARD
  Top 0.305: R27.1 75.57,80.33 R28.2 74.78,80.18 U$6.3 66.69,80.18 55.16,68.66 U1.27
FAULT_2_BMS1_IN  (via drill 0.35)
  Top 0.406: v41.53,6.35 81.4,6.35 85.09,10.03 85.09,76.71 81.47,80.33 R27.2
  Bottom 0.406: 42.66,11.23 D4.C 42.66,17.59 R12.1 40.47,18.1 Q4.1 | R4.2 C2.1 42.86,11.43 42.66,11.23 | U$12.6 17.14,29.61 17.14,11.94 22.86,6.22 40.13,6.22 | 40.13,6.22 41.53,7.62 41.53,10.1 42.66,11.23 | 40.13,6.22 41.41,6.22 v41.53,6.35
FAULT_3_ARD
  Top 0.305: R29.1 75.57,75.25 R30.2 74.78,75.1 U$7.3 62.25,75.1 54.97,67.82 52.4,67.82 U1.26
FAULT_3_BMS2_IN  (via drill 0.35)
  Top 0.406: v56.26,7.03 81.3,7.03 84.53,10.26 84.53,73.03 82.31,75.25 R29.2
  Bottom 0.406: R5.2 C3.1 56.83,11.43 56.63,11.23 | 56.63,11.23 D5.C 56.63,16.51 56.63,16.88 56.63,17.94 56.64,17.95 | U$12.7 16.59,26.17 16.59,11.71 22.63,5.66 53.67,5.66 55.04,7.03 | 55.04,7.03 55.63,7.62 55.63,10.09 56.63,11.1 56.63,11.23 | 55.04,7.03 v56.26,7.03 | Q3.1 56.64,17.95 | 56.64,17.95 57,17.95 R22.1
FAULT_4_ARD
  Top 0.305: R31.1 75.57,70.17 R32.2 74.78,70.02 U$8.3 70.95,69.85 57.65,69.85 54.86,67.06 U1.25
FAULT_4_IMD_IN  (via drill 0.35)
  Top 0.406: v70.23,7.71 81.19,7.71 83.97,10.5 83.97,66.52 80.26,70.23 77.53,70.23 R31.2
  Bottom 0.406: R6.2 C4.1 70.61,11.43 | 70.61,11.43 70.61,11.23 R24.2 69.6,10.09 69.6,8.13 69.18,7.71 | 70.61,11.43 D6.C 70.61,16.88 Q16.1 | U$12.8 16.03,22.73 16.03,11.47 22.4,5.11 66.57,5.11 68.83,7.37 69.18,7.71 | 69.18,7.71 v70.23,7.71
FAULT_RESET
  Bottom 0.406: Q6.1 25.4,28.26 24.76,27.62 R35.2 | Q15.1 Q13.1 Q11.1 Q6.1 | Q6.1 23.03,30.8 R36.2 19.95,30.8 U$12.5
GND  (via drill 0.35)
  Bottom 0.406: 54.78,20.32 55.5,20.32
  other vias: 73.66,83.82 73.66,78.74 73.66,73.66 33.02,77.47 39.37,7.62 39.37,22.86 24.13,7.62 25.4,22.86 45.72,31.75 53.34,22.86 64.77,45.72 58.42,48.26 37.72,36.45 39.37,36.45 68.58,22.86 80.01,22.86 80.01,39.37 68.58,39.37 53.34,39.37 35.56,39.37 53.34,7.62 64.77,8.89 54.86,20.32
  pour Top (isolate 0.254): 0,90.17 0,0 92.71,0 92.71,90.17
  pour Bottom (isolate 0.254): 0,90.17 0,0 92.71,0 92.71,90.17
IMD_FAULT_INDICATOR  (via drill 0.35)
  Top 0.406: v75.95,19.05 76.01,19.11 C14.+ 76.01,25.34 v75.95,25.4 77.22,26.67 | 77.22,26.67 77.47,26.67 U$15.1 | U$15.9 71.07,34.29 v71.25,34.12 | v71.37,32.65 71.68,32.34 71.68,30.1 75.11,26.67 77.22,26.67
  Bottom 0.406: v75.95,19.05 75.95,17.85 R23.1 | v75.95,25.4 D15.C | v71.25,34.12 71.25,32.78 v71.37,32.65
MISO  (via drill 0.35)
  Top 0.305: ISP.1 29.21,77.47 U$9.15 | v34.73,78.23 34.73,75.75 43.42,67.06 U1.16
  Bottom 0.305: v34.73,78.23 34.09,78.87 32.89,78.87 ISP.1
MOSI
  Top 0.305: 34.29,81.9 32.82,80.43 32.82,79.57 32.19,78.94 31.33,78.94 29.27,76.89 26.33,76.89 25.64,76.2 U$9.14 | 34.29,81.9 34.29,82.3 ISP.4 | U1.15 43.28,67.84 35.36,75.77 35.36,80.45 34.29,81.52 34.29,81.9
N$1
  Top 0.305: R1.2 58.1,80.64 DEBUG.2
N$2
  Top 0.813: FUSE.P$1 FUSE.P$4 27.05,47.42 L1.P$1
N$3
  Top 0.406: IC3.7 67.94,55.88 | 67.94,55.88 67.94,55.5 68.28,55.17 71.68,55.17 TCO.TP 75.36,58.85 75.36,58.87 75.87,59.37 U$3.1 | C23.1 60.01,53.98 61.02,54.98 61.02,54.99 R39.1 67.94,55.88
N$4
  Top 0.305: POWER.2 R7.2
N$5
  Top 0.406: U$3.2 75.72,58.42 73.2,55.9 73.2,55.55 72.39,54.74 BCO.TP 68.83,54.61 66.67,52.45 IC3.1 66.46,51.54 R38.1 61.91,46.35 60.9,45.35 60.9,45.34 C22.1
N$6  (via drill 0.35)
  Top 0.406: BRAKE.2 54.25,49.17 54.25,54.99 53.98,55.27 53.98,57.15 55.24,58.42 BTH.TP | v64.99,49.1 65.03,49.15 67.06,49.15 67.77,49.86 67.77,50.07 67.94,50.24 IC3.2
  Bottom 0.406: BRAKE.2 54.59,48.26 55.5,49.17 56.26,49.17 56.33,49.1 v64.99,49.1
N$7  (via drill 0.35)
  Top 0.406: !BSPD_FAULT.TP 44.71,40.4 v45.48,40.4
  Bottom 0.406: R40.2 44.45,41.42 v45.48,40.4 Q1.1 49.01,39.05 U$11.4
N$8  (via drill 0.35)
  Top 0.406: v31.75,15.24 31.75,14.19 BSPD.A
  Bottom 0.406: R11.2 31.75,17.46 v31.75,15.24
N$9  (via drill 0.35)
  Top 0.406: v64.77,24.13 66.04,25.4 v66.04,31.75 | v48.26,35.56 46.99,36.83 U$14.8
  Bottom 0.406: Q4.3 43.35,24.13 v64.77,24.13 | v66.04,31.75 62.23,35.56 v48.26,35.56
N$10
  Top 0.406: R13.1 C18.1 78.74,46.67 78.74,49.53 79.38,50.16 IC1.6 IC1.7
N$11
  Top 0.406: C19.1 80.54,45.93 IC1.5
N$12
  Bottom 0.305: R16.1 19.37,66.67 C12.1
N$13
  Bottom 0.305: C13.1 11.75,65.41 R17.1
N$14
  Bottom 0.305: U$10.8 23.82,75.56 R18.2
N$15
  Bottom 0.406: Q2.1 43.67,39.05 Q1.3 44.45,37.93 44.45,36.83 46.67,34.61 R9.2
N$16  (via drill 0.35)
  Top 0.406: THROTTLE.2 TTH.TP 53.46,58.54 v54.4,58.54 | v69.22,56.39 IC3.6
  Bottom 0.406: v54.4,58.54 67.06,58.54 v69.22,56.39
N$18  (via drill 0.35)
  Top 0.406: v64.77,22.86 67.31,25.4 v67.31,31.75 | v60.96,36.83 U$16.8
  Bottom 0.406: Q3.3 56.05,22.86 v64.77,22.86 | v67.31,31.75 62.23,36.83 v60.96,36.83
N$27
  Top 0.508: U$13.5 37.05,35.56 46.99,35.56 48.26,34.29 U$14.4
N$28  (via drill 0.35)
  Top 0.406: v29.21,29.21 29.21,31.75 U$13.10
  Bottom 0.406: Q6.3 v29.21,29.21
N$31
  Top 0.508: U$14.5 51.02,35.56 60.96,35.56 62.23,34.29 U$16.4
N$32  (via drill 0.35)
  Top 0.406: v27.56,20.32 C16.- 29.4,25.34 v29.34,25.4 28.07,26.67 U$13.12
  Bottom 0.406: Q5.3 26.84,20.32 v27.56,20.32 | v29.34,25.4 D2.A
N$34  (via drill 0.35)
  Top 0.406: v45.72,15.24 45.72,14.19 BMS1.A
  Bottom 0.406: R20.2 46.04,15.56 v45.72,15.24
N$35  (via drill 0.35)
  Top 0.406: v43.18,29.21 43.18,31.75 U$14.10
  Bottom 0.406: Q11.3 v43.18,29.21
N$36
  Top 0.508: U$16.5 64.98,35.56 74.93,35.56 76.2,34.29 U$15.4
N$37  (via drill 0.35)
  Top 0.406: v59.69,15.24 59.69,14.19 BMS2.A
  Bottom 0.406: R21.2 60.01,15.56 v59.69,15.24
N$38  (via drill 0.35)
  Top 0.406: v57.15,29.21 57.15,31.75 U$16.10
  Bottom 0.406: Q13.3 v57.15,29.21
N$42  (via drill 0.35)
  Top 0.406: v73.66,15.24 73.66,14.19 IMD.A
  Bottom 0.406: R23.2 73.98,15.56 v73.66,15.24
N$43  (via drill 0.35)
  Top 0.406: v71.12,29.21 71.12,31.75 U$15.10
  Bottom 0.406: Q15.3 v71.12,29.21
N$44  (via drill 0.35)
  Top 0.406: v69.47,20.19 69.6,20.32 C14.- 71.12,20.51 v71.12,25.4 69.85,26.67 U$15.12
  Bottom 0.406: Q16.3 69.43,20.15 v69.47,20.19 | v71.12,25.4 D15.A
RESET  (via drill 0.35)
  Top 0.305: ISP.5 39.37,82.55 | v54.13,72.87 54.1,72.9 54.1,81.28 52.83,82.55 39.37,82.55 | v54.14,70.95 53.42,70.23 52.4,70.23 U1.29 | 39.37,82.55 36.83,85.09 | 36.83,85.09 36.51,85.41 R15.1 | 36.83,85.09 34.92,85.09 32.82,82.98 32.82,82.11 32.19,81.48 31.32,81.48 29.84,80.01 U$9.17
  Bottom 0.305: v54.13,72.87 v54.14,72.86 v54.14,70.95
RXCAN  (via drill 0.35)
  Top 0.305: U$9.2 v15.75,80.01
  Bottom 0.305: v15.75,80.01 16.38,79.38 U$10.4
SCK
  Top 0.305: ISP.3 33.47,79.18 | 33.47,79.18 32.77,78.49 31.52,78.49 29.46,76.43 26.52,76.43 25.02,74.93 U$9.13 | U1.17 44.7,66.5 43.28,66.5 34.04,75.74 34.04,78.61 33.47,79.18
TXCAN  (via drill 0.35)
  Top 0.305: v15.62,81.28 U$9.1
  Bottom 0.305: U$10.1 17.78,75.56 18.16,75.95 18.16,80.39 17.27,81.28 v15.62,81.28
XTAL1
  Top 0.305: U$1.3 49.23,80.1 | 49.23,80.1 49.64,79.69 C9.1 | U1.7 46.25,74.83 47.94,76.51 47.94,78.37 49.23,79.67 49.23,80.1
XTAL2
  Top 0.305: U1.8 45.47,74.93 44.79,75.61 U$1.1 44.34,77.79 C10.1
~CAN_INT  (via drill 0.35)
  Top 0.305: U1.32 v51.18,72.64 | v25.27,73.65 v25.26,73.66 U$9.12
  Bottom 0.305: v51.18,72.64 26.28,72.64 v25.27,73.65
~CS  (via drill 0.35)
  Top 0.305: U1.9 43.56,73.23 v43.56,73.33 | v25.02,78.74 U$9.16
  Bottom 0.305: v43.56,73.33 31.19,73.33 25.78,78.74 v25.02,78.74

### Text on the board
tNames: IFE 2018 Shutdown Board | V 4.2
